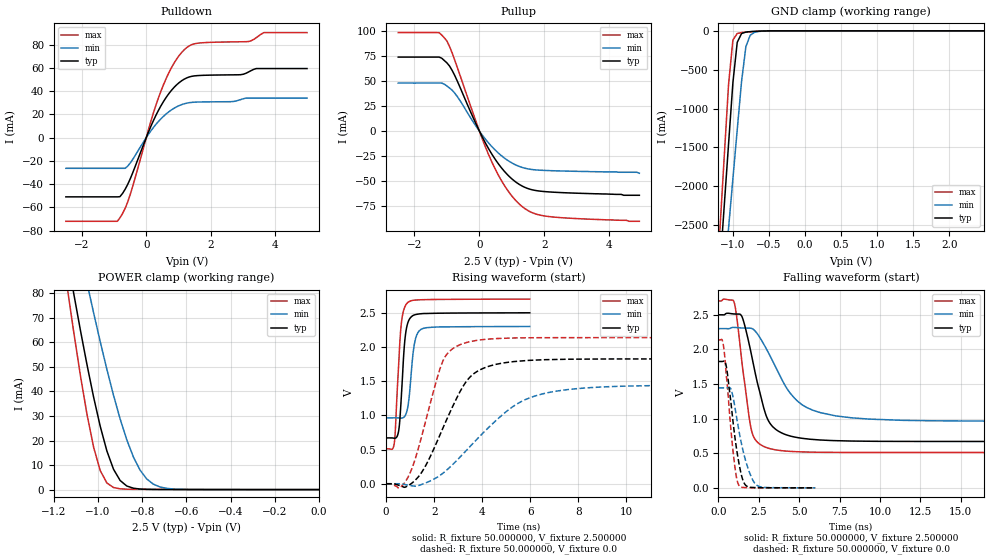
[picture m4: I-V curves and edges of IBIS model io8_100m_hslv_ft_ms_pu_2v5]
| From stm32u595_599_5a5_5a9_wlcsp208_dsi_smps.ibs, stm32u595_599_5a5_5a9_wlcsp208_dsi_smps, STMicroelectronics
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|   Model io8_100m_hslv_ft_ms_pu_2v5
[Model]  io8_100m_hslv_ft_ms_pu_2v5
Model_type I/O
Polarity   Non-Inverting
Enable   Active-Low
Vinl =   0.750000V
Vinh =   1.750000V
Vmeas =  1.250000V
Cref =   50.000000pF
Rref =   100.000000M
Vref =   0.0V
C_comp   3.340900pF   3.338500pF   3.380300pF
[Temperature Range]   25.000000   0.140000k   -40.000000
[Pullup Reference]   2.500000V   2.300000V   2.700000V
[Pulldown Reference]   0.0V   0.0V   0.0V
[POWER Clamp Reference]   2.500000V   2.300000V   2.700000V
[GND Clamp Reference]   0.0V   0.0V   0.0V
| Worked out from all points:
|   slope of the pulldown table from 0 to 0.375 V, typ, clamps not added: 16.1 ohm
|   slope of the pullup table from 0 to 0.375 V, typ, clamps not added: 16.6 ohm
|   GND clamp passes 1 mA (typ) near -0.50 V on its own axis
|   POWER clamp passes 1 mA (typ) near -0.85 V on its own axis
|   rising waveform, R_fixture 50.000000, V_fixture 2.500000: 20-80 % time 199ps typ, 225ps min, 204ps max; typ from 0.671 V to 2.5 V
|   rising waveform, R_fixture 50.000000, V_fixture 0.0: 20-80 % time 1.48ns typ, 2.6ns min, 1ns max; typ from 0.001 V to 1.83 V
|   falling waveform, R_fixture 50.000000, V_fixture 2.500000: 20-80 % time 1.12ns typ, 2.11ns min, 708ps max; typ from 2.5 V to 0.671 V
|   falling waveform, R_fixture 50.000000, V_fixture 0.0: 20-80 % time 608ps typ, 794ps min, 496ps max; typ from 1.83 V to 0.001 V
[Pulldown]
|Voltage   I(typ)   I(min)   I(max)
-2.5V     -51mA      -26.45mA   -72.04mA
-900mV    -51mA      -26.45mA   -72.04mA
-820mV    -50.89mA   -26.45mA   -69.09mA
-500mV    -35.59mA   -21.93mA   -49.09mA
140mV     9.488mA    5.639mA    13.76mA
460mV     27.5mA     16.24mA    40.22mA
860mV     43.07mA    25.18mA    63.88mA
1.26V     51.38mA    29.65mA    77.49mA
1.66V     53.45mA    30.63mA    81.42mA
3.18V     56.44mA    33.99mA    82.68mA
3.66V     59.4mA     33.99mA    90.38mA
5V        59.4mA     33.99mA    90.38mA
[Pullup]
|Voltage   I(typ)   I(min)   I(max)
-2.5V     74.06mA    48.12mA    98.57mA
-1.24V    74.06mA    48.12mA    98.42mA
-1V       68.23mA    45.16mA    90.11mA
-840mV    60.7mA     40.97mA    78.19mA
-680mV    49.98mA    34.52mA    63.57mA
-40mV     2.737mA    1.848mA    3.643mA
360mV     -21.77mA   -14.61mA   -29.22mA
840mV     -42.69mA   -28.49mA   -57.8mA
1.32V     -54.89mA   -36.24mA   -75.42mA
1.64V     -58.66mA   -38.36mA   -81.62mA
2.12V     -60.6mA    -39.32mA   -85.19mA
4.92V     -64mA      -42mA      -90mA
[GND_clamp]
|Voltage   I(typ)   I(min)   I(max)
-2.5V     -9.446A    -9.524A    -9.146A
-1.18V    -3.045A    -3.8A      -2.552A
-1.12V    -2.248A    -3.166A    -1.614A
-1.06V    -1.452A    -2.533A    -685.3mA
-1V       -665mA     -1.901A    -117.9mA
-940mV    -148mA     -1.272A    -34.32mA
-880mV    -35.13mA   -651.5mA   -22.79mA
-820mV    -16mA      -203.9mA   -17.07mA
-760mV    -10.46mA   -56.88mA   -12.26mA
-700mV    -7.068mA   -18.52mA   -8.146mA
-400mV    -103.3uA   -375.9uA   -42.12uA
2.48V     0A         14.84nA    0A
[POWER_clamp]
|Voltage   I(typ)   I(min)   I(max)
-2.49V    881.1mA    773.1mA    1.07A
-1.14V    95.32mA    122.8mA    82.93mA
-1.11V    79.97mA    109.7mA    64.26mA
-1.05V    50.95mA    84.3mA     30.69mA
-1.02V    37.7mA     72.08mA    17.29mA
-990mV    25.79mA    60.29mA    7.738mA
-930mV    8.312mA    38.47mA    853.6uA
-900mV    3.712mA    28.81mA    314.2uA
-840mV    566.7uA    13.29mA    124.4uA
-780mV    119.5uA    4.365mA    94.68uA
-660mV    39.4uA     251.7uA    58.31uA
0V        0A         18.89nA    0A
[Ramp]
| variable   typ   min   max
dV/dt_r  1.09488/1.47405n   0.86569/2.59936n   1.28167/1.00228n
dV/dt_f  1.09764/1.11746n   0.80162/2.10128n   1.31315/0.70718n
R_load = 50.000000
[Rising Waveform]
R_fixture= 50.000000
V_fixture= 2.500000
V_fixture_min= 2.300000
V_fixture_max= 2.700000
|time   V(typ)   V(min)   V(max)
0s        670.5mV    963.9mV    511.4mV
336.3ps   666.3mV    964.2mV    587.4mV
384.4ps   667.6mV    964.1mV    795.4mV
516.5ps   765.5mV    963.4mV    1.714V
648.6ps   1.373V     960.9mV    2.389V
756.8ps   2.012V     979mV      2.567V
876.9ps   2.321V     1.08V      2.642V
1.177ns   2.469V     2.045V     2.686V
1.453ns   2.487V     2.258V     2.691V
5.982ns   2.5V       2.3V       2.7V
[Rising Waveform]
R_fixture= 50.000000
V_fixture= 0.0
V_fixture_min= 0.0
V_fixture_max= 0.0
|time   V(typ)   V(min)   V(max)
0s        601.7uV    748.1uV    547.5uV
750.8ps   -51.86mV   -8.964mV   6.498mV
1.051ns   3.866mV    -27.41mV   203.7mV
1.401ns   128.1mV    -19.42mV   593.1mV
2.402ns   844.7mV    165mV      1.824V
3.453ns   1.546V     529.6mV    2.075V
4.154ns   1.703V     784mV      2.113V
5.405ns   1.789V     1.157V     2.133V
7.508ns   1.821V     1.375V     2.137V
24.92ns   1.826V     1.444V     2.137V
[Falling Waveform]
R_fixture= 50.000000
V_fixture= 2.500000
V_fixture_min= 2.300000
V_fixture_max= 2.700000
|time   V(typ)   V(min)   V(max)
0s        2.5V       2.3V       2.7V
951ps     2.512V     2.318V     2.693V
1.151ns   2.511V     2.315V     2.426V
1.451ns   2.475V     2.309V     1.812V
2.052ns   1.909V     2.304V     821.5mV
2.953ns   1.042V     2.012V     583.8mV
3.554ns   843.4mV    1.737V     548.4mV
4.855ns   727.9mV    1.261V     522.7mV
7.257ns   682.2mV    1.04V      513mV
24.92ns   670.5mV    963.9mV    511.4mV
[Falling Waveform]
R_fixture= 50.000000
V_fixture= 0.0
V_fixture_min= 0.0
V_fixture_max= 0.0
|time   V(typ)   V(min)   V(max)
0s        1.826V     1.444V     2.137V
264.3ps   1.827V     1.444V     2.107V
468.5ps   1.773V     1.444V     1.668V
744.7ps   1.284V     1.438V     905.9mV
948.9ps   856.9mV    1.253V     429.4mV
1.105ns   583mV      1.043V     162mV
1.261ns   361.4mV    829.9mV    38.33mV
1.646ns   48.04mV    421.9mV    4.708mV
2.402ns   3.773mV    33.05mV    2.188mV
5.982ns   601.7uV    748.1uV    547.5uV
